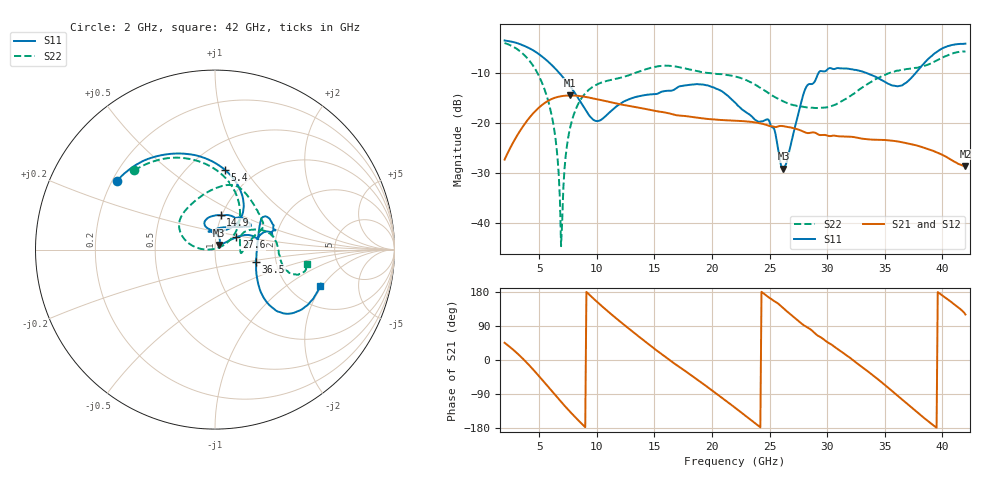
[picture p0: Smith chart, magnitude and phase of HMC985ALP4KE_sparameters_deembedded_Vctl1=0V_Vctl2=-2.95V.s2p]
!s2p File: Measurements: S11, S21, S12, S22
# GHz S dB R 50.0
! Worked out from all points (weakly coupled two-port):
!   401 points, 2 GHz to 42 GHz, reference 50 ohm
!   highest |S21| = -14.52 dB at 7.7 GHz (marker M1); lowest = -28.7 dB at 42 GHz (marker M2)
!   lowest |S11| = -29.2 dB at 26.2 GHz (marker M3), VSWR 1.07, Z = 52.3 + j2.74 ohm
!   |S11| at or under -10 dB: 6.743 GHz to 29.26 GHz (22.51 GHz wide, 125 % of centre); 33.39 GHz to 37.7 GHz (4.305 GHz wide, 12.1 % of centre)
!   |S22| runs from -44.7 to -4.0 dB; largest |S21 - S12| = 0.00072
!   S11 on the Smith chart (normalised r, x): 2 GHz: 0.22, +0.30; 5.4 GHz: 0.74, +0.82; 14.9 GHz: 0.99, +0.39; 27.6 GHz: 1.26, +0.18; 36.5 GHz: 1.57, -0.22; 42 GHz: 2.92, -1.90
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2  -3.50 145.2  -27.35 45.4  -27.33 45.4  -4.02 135.6
3.5  -4.39 119.2  -21.04 6.0  -21.04 6.0  -5.99 100.8
5.4  -7.00 82.8  -16.15 -57.2  -16.16 -57.2  -12.87 52.4
6.3  -8.91 66.8  -15.03 -89.3  -15.02 -89.3  -21.25 31.1
6.9  -10.41 58.0  -14.67 -110.3  -14.69 -110.3  -44.68 70.1
7.1  -10.95 55.7  -14.60 -117.1  -14.62 -117.2  -32.99 177.4
7.7  -12.70 51.0  -14.52 -137.1  -14.50 -137.1  -20.86 175.5
8.7  -16.23 53.1  -14.68 -168.4  -14.70 -168.4  -14.98 161.5
10.1  -19.63 88.2  -15.30 151.4  -15.27 151.4  -12.21 144.8
14.9  -14.27 80.4  -17.50 32.2  -17.50 32.2  -8.86 81.8
15.4  -14.02 74.3  -17.74 20.9  -17.78 20.8  -8.64 77.2
19.3  -12.36 33.7  -19.13 -64.4  -19.15 -64.4  -9.87 42.6
22  -15.92 52.1  -19.56 -125.7  -19.57 -125.8  -10.71 24.4
25  -19.77 99.5  -20.63 163.9  -20.62 163.9  -14.19 12.5
26.2  -29.17 48.9  -20.66 136.5  -20.67 136.5  -15.71 0.7
27.6  -17.21 30.0  -21.42 100.4  -21.45 100.4  -16.64 -7.5
28.7  -12.20 13.0  -21.91 77.2  -21.88 77.2  -16.96 -2.9
31  -9.06 23.2  -22.69 27.0  -22.67 27.0  -15.99 26.3
35.4  -12.26 11.8  -23.50 -75.8  -23.50 -75.8  -10.05 16.9
36.5  -12.51 -16.5  -23.88 -104.1  -23.88 -104.2  -9.36 9.4
39.6  -5.67 -43.0  -25.98 179.2  -25.98 179.0  -7.42 -16.9
42  -4.15 -18.8  -28.65 120.1  -28.67 120.2  -5.68 -9.0
